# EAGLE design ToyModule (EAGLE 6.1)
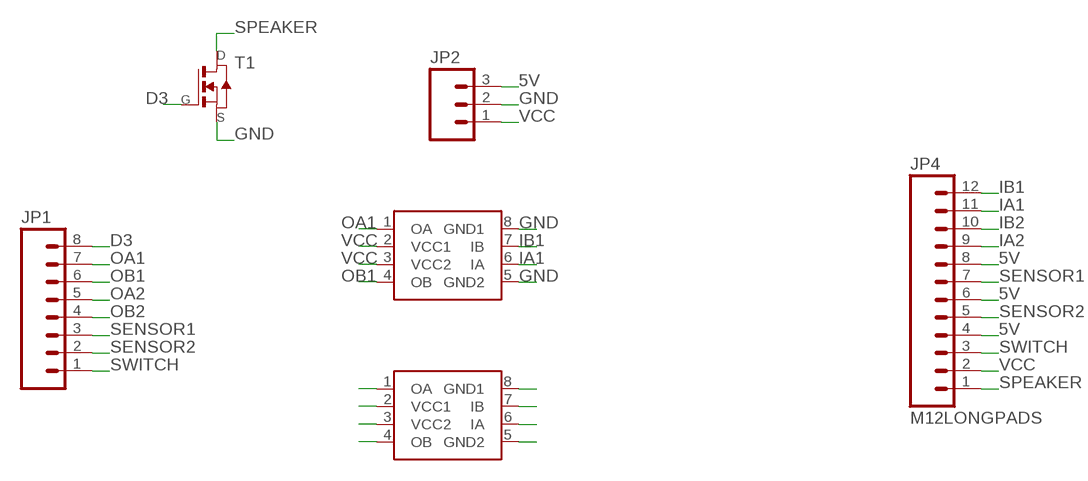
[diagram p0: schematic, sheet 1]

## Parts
JP1  M08LONGPADS  [1X08_LONGPADS]
JP2  M03LONGPADS  [1X03_LONGPADS]
JP4  M12LONGPADS  [1X12_LONGPADS]
T1  NMOSFETSOT23  [SOT-23]
U$1  L9110  L9110_SOP8  [SOIC8]
U$2  L9110_SOP8  [SOIC8]

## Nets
5V: JP2.3 JP4.4 JP4.6 JP4.8
D3: JP1.8 T1.3(G)
GND: JP2.2 T1.2(S) U$1.5(GND2) U$1.8(GND1) U$2.5(GND2) U$2.8(GND1)
IA1: JP4.11 U$1.6(IA)
IA2: JP4.9 U$2.6(IA)
IB1: JP4.12 U$1.7(IB)
IB2: JP4.10 U$2.7(IB)
OA1: JP1.7 U$1.1(OA)
OA2: JP1.5 U$2.1(OA)
OB1: JP1.6 U$1.4(OB)
OB2: JP1.4 U$2.4(OB)
SENSOR1: JP1.3 JP4.7
SENSOR2: JP1.2 JP4.5
SPEAKER: JP4.1 T1.1(D)
SWITCH: JP1.1 JP4.3
VCC: JP2.1 JP4.2 U$1.2(VCC1) U$1.3(VCC2) U$2.2(VCC1) U$2.3(VCC2)

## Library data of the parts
JP1 = SparkFun-Connectors:M08: Header 8 Standard 8-pin 0.1" header. Use with straight break away headers (SKU : PRT-00116), right angle break away headers (PRT-00553), swiss pins (PRT-00743), machine pins (PRT-00117), and female headers (PRT-00115).
JP2 = SparkFun-Connectors:M03: Header 3 Standard 3-pin 0.1" header. Use with straight break away headers (SKU : PRT-00116), right angle break away headers (PRT-00553), swiss pins (PRT-00743), machine pins (PRT-00117), and female headers (PRT-00115). Molex polarized connector foot print use with SKU : PRT-08232 with associated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
JP4 = SparkFun-Connectors:M12: Header 12 Standard 12-pin 0.1" header. Use with straight break away headers (SKU : PRT-00116), right angle break away headers (PRT-00553), swiss pins (PRT-00743), machine pins (PRT-00117), and female headers (PRT-00115).
T1 = fab:NMOSFET: MOS FET
U$1 U$2 = fab:L9110_SOP8

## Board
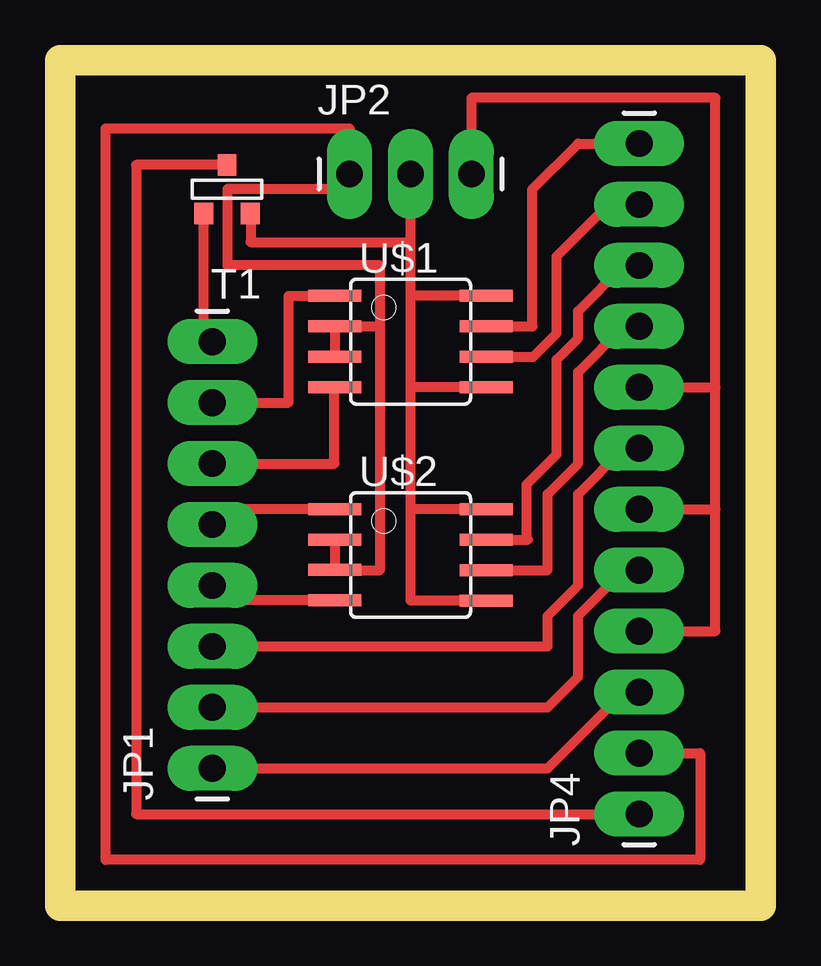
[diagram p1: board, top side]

Size 29.19 x 35.23 mm. Coordinates in mm from the lower left corner, seen from the top.
Outline: 0,0 29.19,0 29.19,35.23 0,35.23 0,0
Copper layers (1*16): Top 0.035mm / dielectric 1.5mm / Bottom 0.035mm
Design rules: minimum track width 10mil, minimum drill 24mil, track to track 8mil, track to pad 8mil, pad to pad 8mil, via to via 8mil, smd to smd 8mil, copper to edge 40mil, drill to drill 8mil, minimum pad ring 10mil, minimum via ring 8mil, stop-mask expansion 4mil, vias tented up to drill 0mil, thermal gap 10mil

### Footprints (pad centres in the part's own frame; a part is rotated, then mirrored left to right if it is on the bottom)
1X08_LONGPADS = drill 1.118 pad 1.88 long: 1 0,0; 2 2.54,0; 3 5.08,0; 4 7.62,0; 5 10.16,0; 6 12.7,0; 7 15.24,0; 8 17.78,0
1X03_LONGPADS = drill 1.118 pad 1.88 long: 1 0,0; 2 2.54,0; 3 5.08,0
1X12_LONGPADS = drill 1.118 pad 1.88 long: 1 0,0; 2 2.54,0; 3 5.08,0; 4 7.62,0; 5 10.16,0; 6 12.7,0; 7 15.24,0; 8 17.78,0; 9 20.32,0; 10 22.86,0; 11 25.4,0; 12 27.94,0
SOT-23 = smd 0.787 x 0.889: 1 0.025,-1.016; 2 -0.94,1.016; 3 0.991,1.016
SOIC8 = smd 0.5 x 2.2: 1 -1.905,-3.154; 2 -0.645,-3.154; 3 0.625,-3.154; 4 1.895,-3.154; 5 1.905,3.154; 6 0.635,3.154; 7 -0.635,3.154; 8 -1.905,3.154

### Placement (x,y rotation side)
JP1  6.35,5.71 90 top
JP2  12.06,30.48 0 top
JP4  24.13,3.81 90 top
T1  6.99,29.84 180 top
U$1  14.61,23.5 270 top
U$2  14.61,14.61 270 top

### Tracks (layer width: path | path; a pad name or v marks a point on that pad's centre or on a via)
5V
  Top 0.406: JP4.8 27.3,21.59 | 27.3,21.59 27.3,33.66 17.14,33.66 JP2.3 | JP4.4 27.3,11.43 27.3,16.51 | 27.3,16.51 27.3,21.59 | JP4.6 27.3,16.51
D3
  Top 0.406: JP1.8 5.99,23.5 T1.3
GND
  Top 0.406: U$2.5 14.61,12.7 14.61,16.51 | 14.61,16.51 14.61,21.59 | 14.61,25.4 14.61,27.64 | 14.61,27.64 JP2.2 | U$1.8 14.61,25.4 | T1.2 7.95,28.83 7.95,27.64 14.61,27.64 | U$1.5 14.61,21.59 | 14.61,21.59 14.61,25.4 | U$2.8 14.61,16.51
IA1
  Top 0.406: U$1.6 19.71,22.86 20.7,23.84 20.7,27.05 22.86,29.21 JP4.11
IA2
  Top 0.406: U$2.6 20.32,13.97 20.32,17.14 21.59,18.41 21.59,22.23 23.5,24.13 JP4.9
IB1
  Top 0.406: U$1.7 19.68,24.13 19.68,29.84 21.59,31.75 JP4.12
IB2
  Top 0.406: U$2.7 19.5,15.24 19.45,15.29 19.45,17.55 20.7,18.8 20.7,22.75 21.59,23.64 21.59,24.77 23.5,26.67 JP4.10
OA1
  Top 0.406: JP1.7 9.53,20.95 9.53,25.4 U$1.1
OA2
  Top 0.406: U$2.1 6.99,16.51 JP1.5
OB1  (1 unrouted)
  Top 0.406: JP1.6 11.43,18.41 11.43,21.59
OB2
  Top 0.406: U$2.4 6.97,12.71 JP1.4
SENSOR1
  Top 0.406: JP1.3 20.32,10.79 20.32,12.06 21.59,13.34 21.59,17.14 23.5,19.05 JP4.7
SENSOR2
  Top 0.406: JP1.2 20.32,8.26 21.59,9.53 21.59,12.06 23.5,13.97 JP4.5
SPEAKER
  Top 0.406: T1.1 3.17,30.86 3.17,3.81 JP4.1
SWITCH
  Top 0.406: JP1.1 20.32,5.71 23.5,8.89 JP4.3
VCC
  Top 0.406: U$1.2 U$1.3 | 13.34,24.13 13.34,13.97 11.46,13.97 U$2.3 U$2.2 | U$1.2 11.46,24.13 13.34,24.13 | U$1.2 13.34,24.14 | 13.34,24.14 13.34,24.13 | 13.34,24.14 13.34,26.67 6.99,26.67 6.99,29.84 12.06,29.84 JP2.1 12.06,32.38 1.91,32.38 1.91,1.91 26.67,1.91 26.67,6.35 JP4.2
